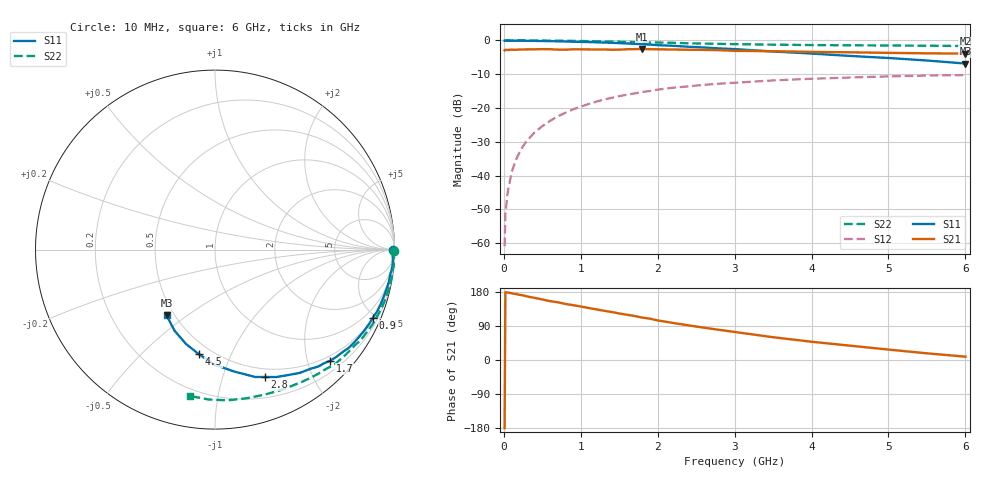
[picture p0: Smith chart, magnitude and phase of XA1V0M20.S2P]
! SIEMENS Discrete & RF Semiconductors
! BFY180
! Si NPN RF Bipolar Junction Transistor in MICRO-X
! VCE = 1 V  IC = 0.2 mA
! Common Emitter S-Parameters:  May  1997
# GHz  S  MA  R  50
!  f  S11  S21  S12  S22
! GHz  MAG  ANG  MAG  ANG  MAG  ANG  MAG  ANG
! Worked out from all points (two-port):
!   36 points, 10 MHz to 6 GHz, reference 50 ohm
!   highest |S21| = -2.52 dB at 1.8 GHz (marker M1); lowest = -3.9 dB at 6 GHz (marker M2)
!   |S21| within 3 dB of the highest: start of sweep to end of sweep
!   lowest |S11| = -6.8 dB at 6 GHz (marker M3), VSWR 2.67, Z = 22.7 - j21 ohm
!   |S11| at or under -10 dB: nowhere
!   |S22| runs from -1.6 to 0.0 dB; largest |S21 - S12| = 0.74
!   S11 on the Smith chart (normalised r, x): 10 MHz: open; 900 MHz: 0.52, -4.77; 1.7 GHz: 0.40, -2.42; 2.8 GHz: 0.41, -1.39; 4.5 GHz: 0.43, -0.76; 6 GHz: 0.45, -0.42
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0.01  0.9922 -0.1  0.713 -179.9  0.0009 91.5  0.999 -0.3
0.02  0.9925 -0.7  0.729 178.9  0.0027 89.1  0.9999 -0.4
0.05  0.9896 -1.3  0.721 178.1  0.0056 88.5  0.9995 -1.0
0.1  0.9914 -2.5  0.731 176.2  0.011 87.8  0.9963 -2.1
0.15  0.993 -4.1  0.727 174.3  0.0164 86.7  0.9999 -3.1
0.2  0.9925 -5.2  0.733 172.1  0.0216 85.7  0.9992 -4.2
0.25  0.9898 -6.9  0.736 170.6  0.0273 84.8  1 -5.3
0.3  0.9865 -7.9  0.737 167.8  0.0326 83.3  0.9976 -6.3
0.4  0.9851 -10.6  0.739 163.9  0.0436 81.0  0.9975 -8.3
0.6  0.9758 -15.6  0.742 155.3  0.0644 76.7  0.9929 -12.5
0.9  0.9577 -23.4  0.74 144.7  0.0955 69.2  0.9843 -18.8
1.1  0.9466 -28.5  0.737 137.3  0.1144 65.0  0.9757 -22.8
1.3  0.9324 -33.7  0.735 130.0  0.133 60.3  0.9672 -26.9
1.7  0.8921 -44.0  0.744 116.2  0.1645 51.9  0.9436 -34.6
1.8  0.8768 -46.3  0.748 111.8  0.1722 50.1  0.9393 -36.4
2.2  0.8336 -55.5  0.734 97.8  0.1997 42.1  0.9234 -43.8
2.8  0.7624 -68.5  0.718 79.6  0.2291 31.9  0.8906 -53.4
3.5  0.6864 -81.3  0.693 60.1  0.2561 21.8  0.8669 -63.7
4  0.6399 -90.4  0.677 48.2  0.2707 14.9  0.8546 -70.8
4.5  0.5899 -98.7  0.668 37.8  0.2829 8.7  0.847 -78.0
5.5  0.5049 -116.5  0.645 17.6  0.3022 -3.3  0.8358 -92.5
6  0.4552 -126.4  0.639 8.8  0.3077 -9.5  0.8274 -99.7
